(* Logix 5000 AddOnInstructionDefinition export Banner_S15C_B21_Param_v4; software revision 33.00; part 2 of 2 *)
(* tags used below, declared in another part *)
   S15C : Banner_S15C_B21_v4;
   Port_Data : Banner_IOL_Port_v4;
   Port : DINT;
   Local_Control : DINT;
   Command_Being_Processed : BOOL;
   Index_Write_Inprocess : INT;
   Index_Write_Control : INT;
   Update_Archive : BOOL;
   Inprocess_Index : DINT;
(* Banner_S15C_B21_Param_v4, continued *)

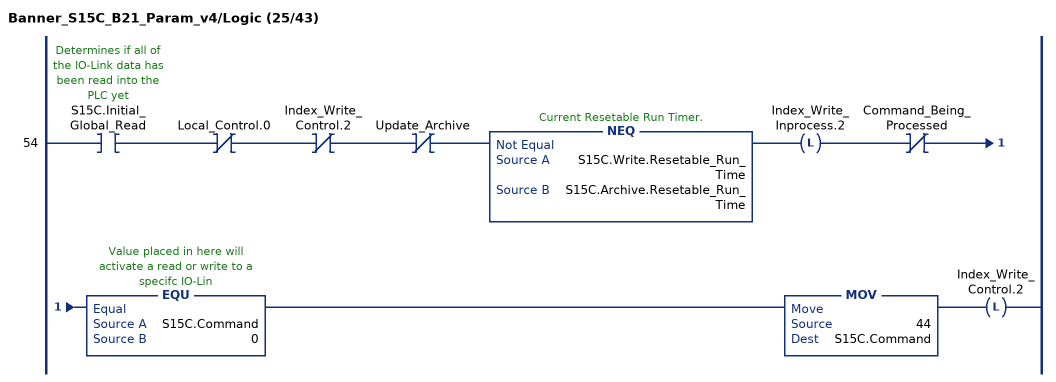
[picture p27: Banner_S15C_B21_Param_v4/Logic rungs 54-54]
   54: XIC(S15C.Initial_Global_Read)XIO(Local_Control.0)XIO(Index_Write_Control.2)XIO(Update_Archive)NEQ(S15C.Write.Resetable_Run_Time,S15C.Archive.Resetable_Run_Time)OTL(Index_Write_Inprocess.2)XIO(Command_Being_Processed)EQU(S15C.Command,0)MOV(44,S15C.Command)OTL(Index_Write_Control.2);
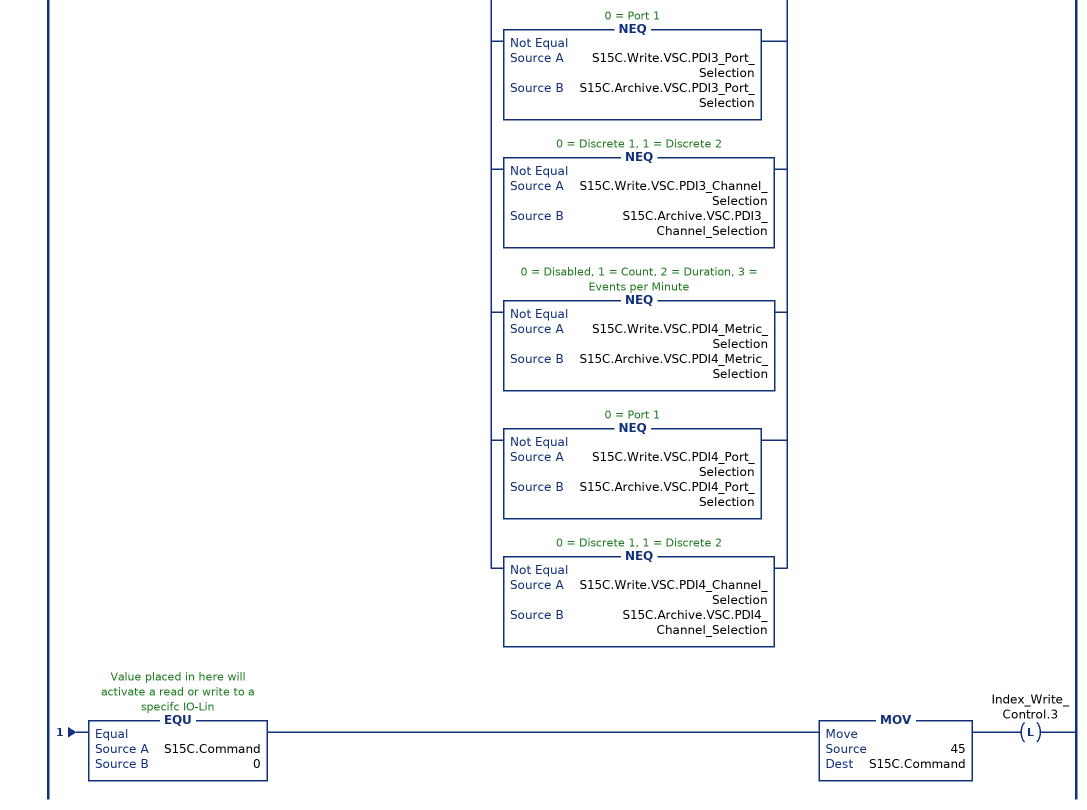
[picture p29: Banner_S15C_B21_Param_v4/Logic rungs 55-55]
   55: XIC(S15C.Initial_Global_Read)XIO(Local_Control.0)XIO(Index_Write_Control.3)XIO(Update_Archive)[NEQ(S15C.Write.VSC.PDI1_Metric_Selection,S15C.Archive.VSC.PDI1_Metric_Selection) ,NEQ(S15C.Write.VSC.PDI1_Port_Selection,S15C.Archive.VSC.PDI1_Port_Selection) ,NEQ(S15C.Write.VSC.PDI1_Channel_Selection,S15C.Archive.VSC.PDI1_Channel_Selection) ,NEQ(S15C.Write.VSC.PDI2_Metric_Selection,S15C.Archive.VSC.PDI2_Metric_Selection) ,NEQ(S15C.Write.VSC.PDI2_Port_Selection,S15C.Archive.VSC.PDI2_Port_Selection) ,NEQ(S15C.Write.VSC.PDI2_Channel_Selection,S15C.Archive.VSC.PDI2_Channel_Selection) ,NEQ(S15C.Write.VSC.PDI3_Metric_Selection,S15C.Archive.VSC.PDI3_Metric_Selection) ,NEQ(S15C.Write.VSC.PDI3_Port_Selection,S15C.Archive.VSC.PDI3_Port_Selection) ,NEQ(S15C.Write.VSC.PDI3_Channel_Selection,S15C.Archive.VSC.PDI3_Channel_Selection) ,NEQ(S15C.Write.VSC.PDI4_Metric_Selection,S15C.Archive.VSC.PDI4_Metric_Selection) ,NEQ(S15C.Write.VSC.PDI4_Port_Selection,S15C.Archive.VSC.PDI4_Port_Selection) ,NEQ(S15C.Write.VSC.PDI4_Channel_Selection,S15C.Archive.VSC.PDI4_Channel_Selection) ]OTL(Index_Write_Inprocess.3)XIO(Command_Being_Processed)EQU(S15C.Command,0)MOV(45,S15C.Command)OTL(Index_Write_Control.3);
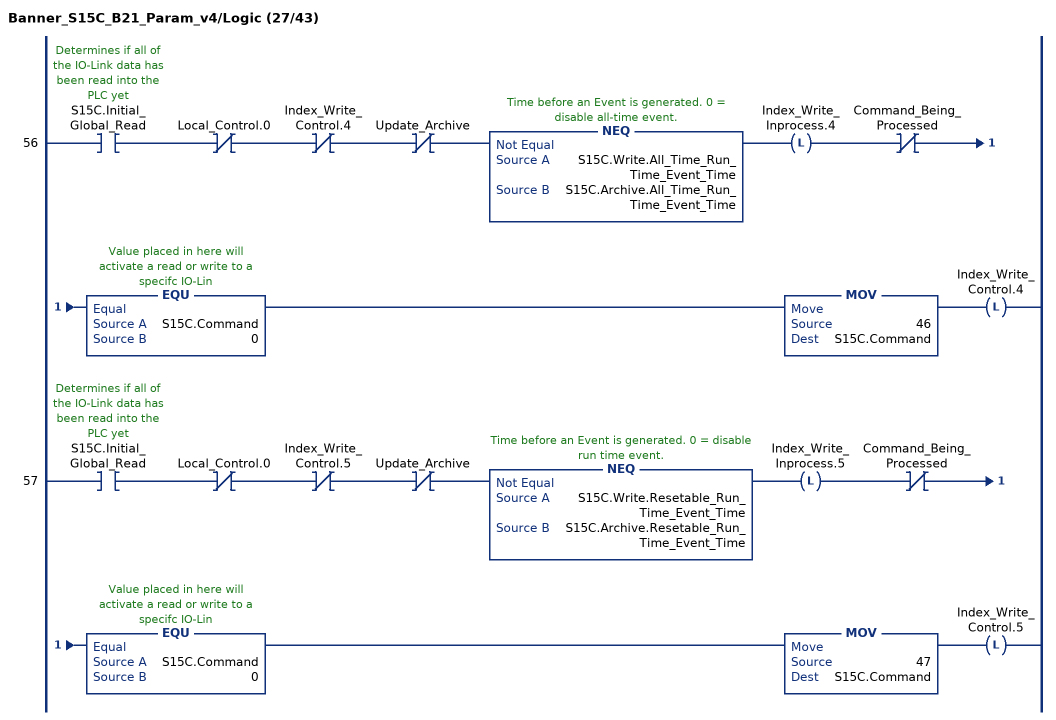
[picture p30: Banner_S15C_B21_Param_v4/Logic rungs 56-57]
   56: XIC(S15C.Initial_Global_Read)XIO(Local_Control.0)XIO(Index_Write_Control.4)XIO(Update_Archive)NEQ(S15C.Write.All_Time_Run_Time_Event_Time,S15C.Archive.All_Time_Run_Time_Event_Time)OTL(Index_Write_Inprocess.4)XIO(Command_Being_Processed)EQU(S15C.Command,0)MOV(46,S15C.Command)OTL(Index_Write_Control.4);
   57: XIC(S15C.Initial_Global_Read)XIO(Local_Control.0)XIO(Index_Write_Control.5)XIO(Update_Archive)NEQ(S15C.Write.Resetable_Run_Time_Event_Time,S15C.Archive.Resetable_Run_Time_Event_Time)OTL(Index_Write_Inprocess.5)XIO(Command_Being_Processed)EQU(S15C.Command,0)MOV(47,S15C.Command)OTL(Index_Write_Control.5);
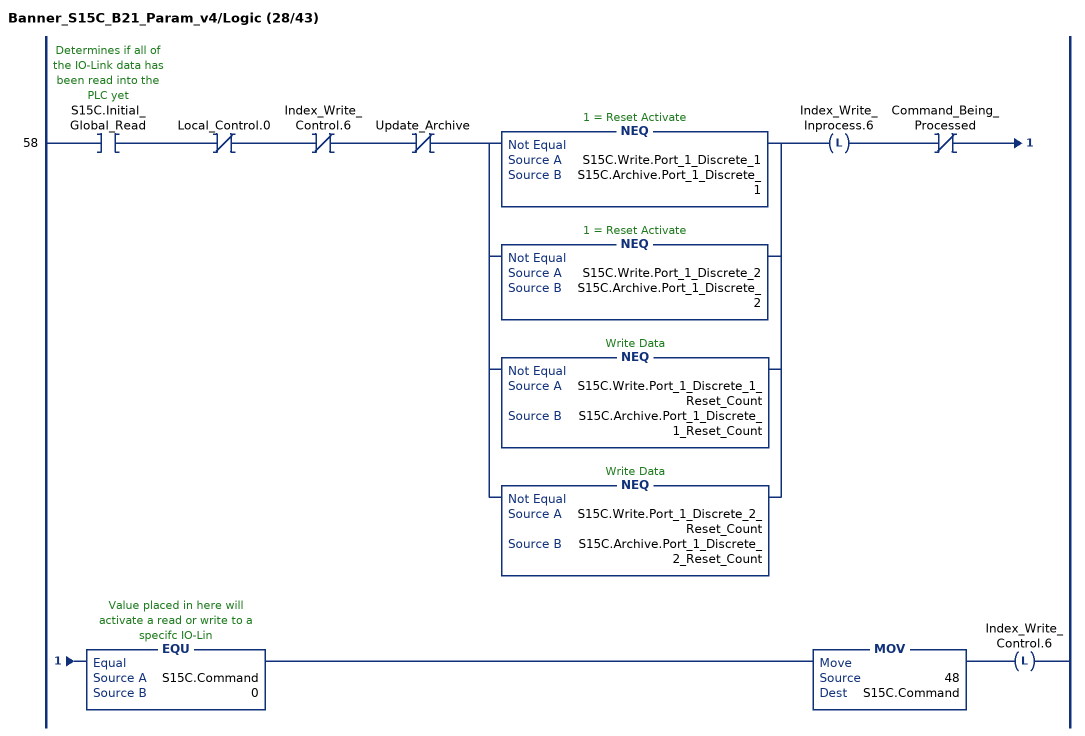
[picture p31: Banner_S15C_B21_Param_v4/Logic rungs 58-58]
   58: XIC(S15C.Initial_Global_Read)XIO(Local_Control.0)XIO(Index_Write_Control.6)XIO(Update_Archive)[NEQ(S15C.Write.Port_1_Discrete_1,S15C.Archive.Port_1_Discrete_1) ,NEQ(S15C.Write.Port_1_Discrete_2,S15C.Archive.Port_1_Discrete_2) ,NEQ(S15C.Write.Port_1_Discrete_1_Reset_Count,S15C.Archive.Port_1_Discrete_1_Reset_Count) ,NEQ(S15C.Write.Port_1_Discrete_2_Reset_Count,S15C.Archive.Port_1_Discrete_2_Reset_Count) ]OTL(Index_Write_Inprocess.6)XIO(Command_Being_Processed)EQU(S15C.Command,0)MOV(48,S15C.Command)OTL(Index_Write_Control.6);
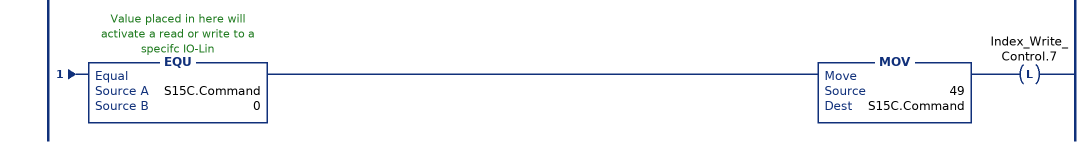
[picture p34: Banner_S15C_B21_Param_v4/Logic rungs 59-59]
   59: XIC(S15C.Initial_Global_Read)XIO(Local_Control.0)XIO(Index_Write_Control.7)XIO(Update_Archive)[NEQ(S15C.Write.Port_1_Configuration.DI1_IO_Selection,S15C.Archive.Port_1_Configuration.DI1_IO_Selection) ,NEQ(S15C.Write.Port_1_Configuration.DI1_Delay_Mode,S15C.Archive.Port_1_Configuration.DI1_Delay_Mode) ,NEQ(S15C.Write.Port_1_Configuration.DI1_Delay_Timer_1,S15C.Archive.Port_1_Configuration.DI1_Delay_Timer_1) ,NEQ(S15C.Write.Port_1_Configuration.DI1_Delay_Timer_2,S15C.Archive.Port_1_Configuration.DI1_Delay_Timer_2) ,NEQ(S15C.Write.Port_1_Configuration.DI2_IO_Selection,S15C.Archive.Port_1_Configuration.DI2_IO_Selection) ,NEQ(S15C.Write.Port_1_Configuration.DI2_Delay_Mode,S15C.Archive.Port_1_Configuration.DI2_Delay_Mode) ,NEQ(S15C.Write.Port_1_Configuration.DI2_Delay_Timer_1,S15C.Archive.Port_1_Configuration.DI2_Delay_Timer_1) ,NEQ(S15C.Write.Port_1_Configuration.DI2_Delay_Timer_2,S15C.Archive.Port_1_Configuration.DI2_Delay_Timer_2) ,NEQ(S15C.Write.Port_1_Configuration.Mirroring_Enable,S15C.Archive.Port_1_Configuration.Mirroring_Enable) ,NEQ(S15C.Write.Port_1_Configuration.Mirroring_Port_Selection,S15C.Archive.Port_1_Configuration.Mirroring_Port_Selection) ,NEQ(S15C.Write.Port_1_Configuration.Mirroring_Channel_Selection,S15C.Archive.Port_1_Configuration.Mirroring_Channel_Selection) ,NEQ(S15C.Write.Port_1_Configuration.Mirroring_Inversion,S15C.Archive.Port_1_Configuration.Mirroring_Inversion) ,NEQ(S15C.Write.Port_1_Configuration.Counts_per_Minute_Mode,S15C.Archive.Port_1_Configuration.Counts_per_Minute_Mode) ]OTL(Index_Write_Inprocess.7)XIO(Command_Being_Processed)EQU(S15C.Command,0)MOV(49,S15C.Command)OTL(Index_Write_Control.7);
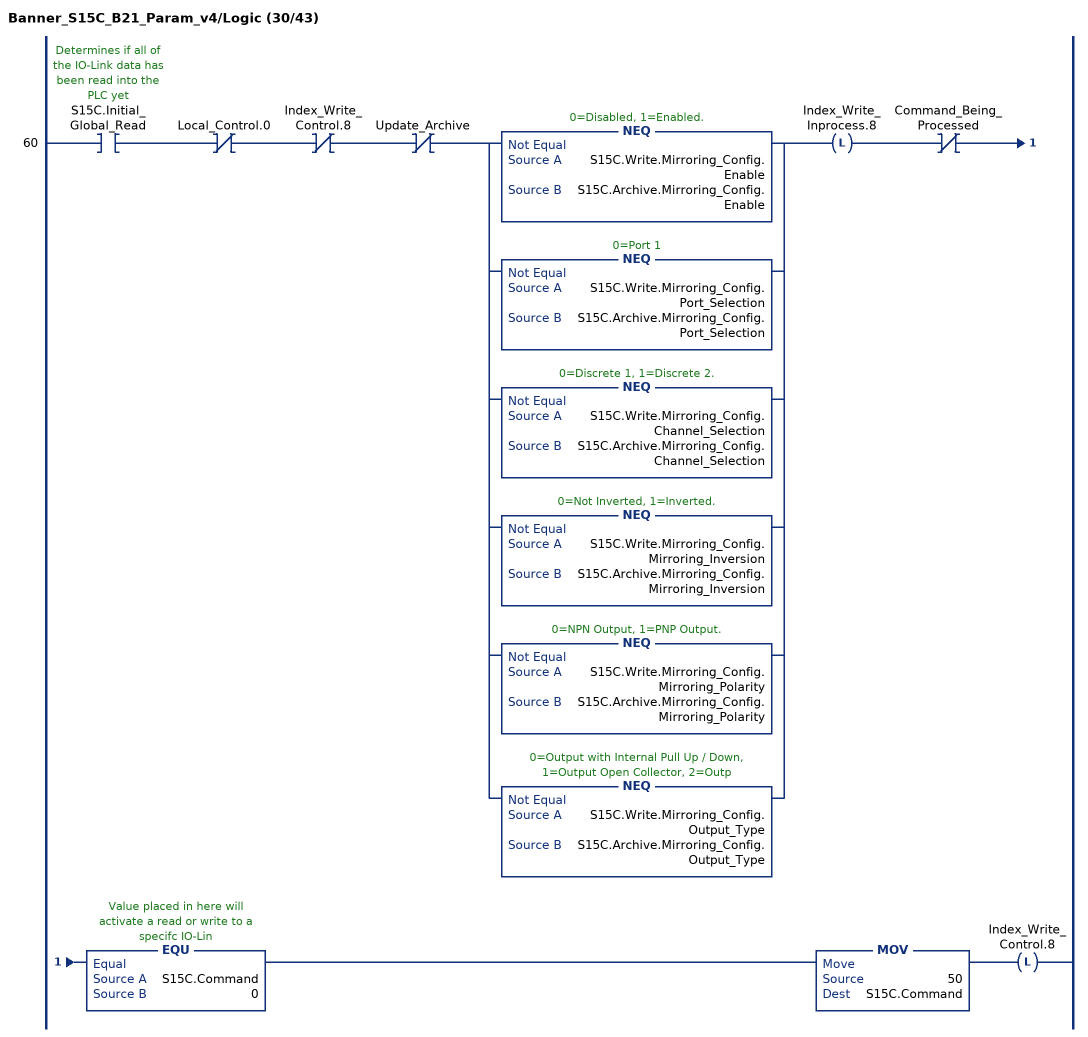
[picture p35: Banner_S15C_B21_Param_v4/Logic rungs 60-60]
   60: XIC(S15C.Initial_Global_Read)XIO(Local_Control.0)XIO(Index_Write_Control.8)XIO(Update_Archive)[NEQ(S15C.Write.Mirroring_Config.Enable,S15C.Archive.Mirroring_Config.Enable) ,NEQ(S15C.Write.Mirroring_Config.Port_Selection,S15C.Archive.Mirroring_Config.Port_Selection) ,NEQ(S15C.Write.Mirroring_Config.Channel_Selection,S15C.Archive.Mirroring_Config.Channel_Selection) ,NEQ(S15C.Write.Mirroring_Config.Mirroring_Inversion,S15C.Archive.Mirroring_Config.Mirroring_Inversion) ,NEQ(S15C.Write.Mirroring_Config.Mirroring_Polarity,S15C.Archive.Mirroring_Config.Mirroring_Polarity) ,NEQ(S15C.Write.Mirroring_Config.Output_Type,S15C.Archive.Mirroring_Config.Output_Type) ]OTL(Index_Write_Inprocess.8)XIO(Command_Being_Processed)EQU(S15C.Command,0)MOV(50,S15C.Command)OTL(Index_Write_Control.8);
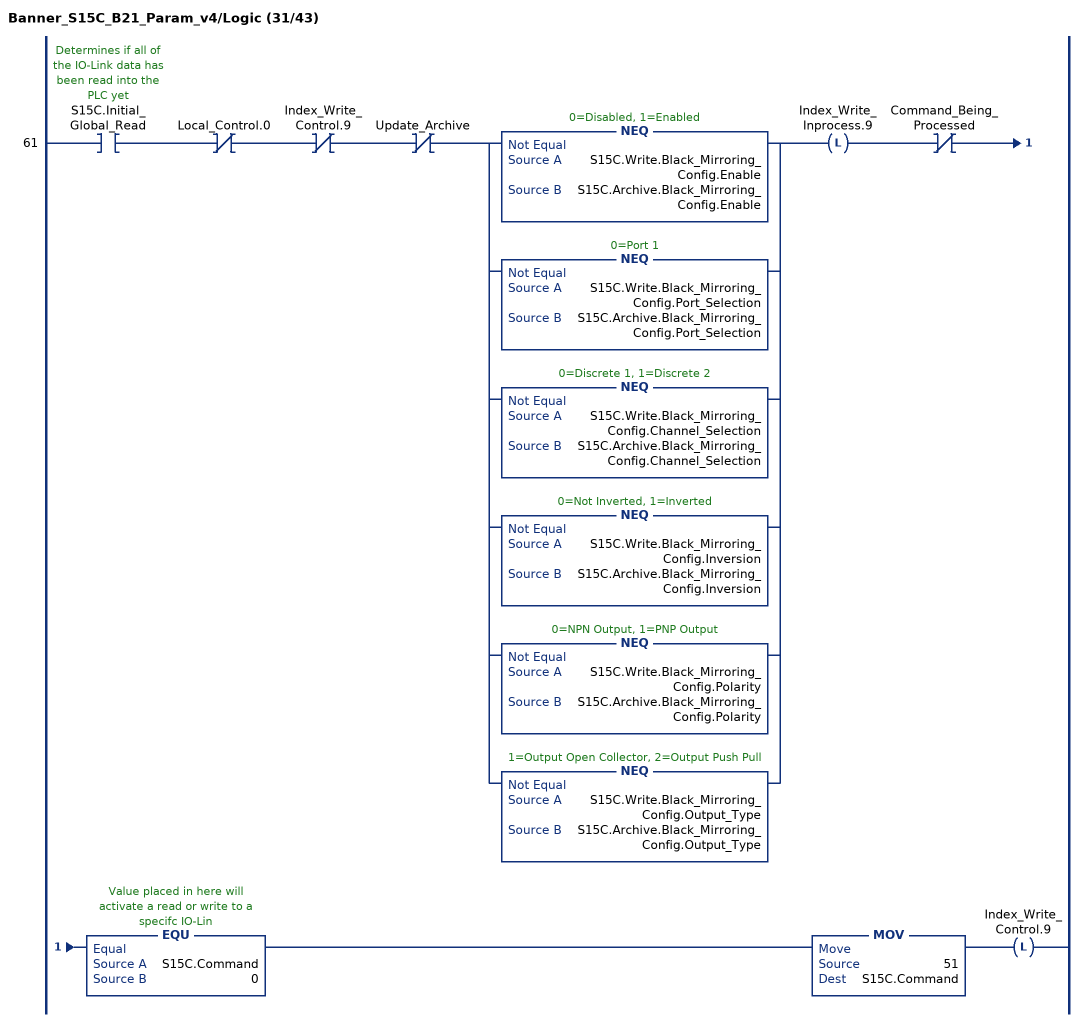
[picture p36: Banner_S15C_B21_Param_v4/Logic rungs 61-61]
   61: XIC(S15C.Initial_Global_Read)XIO(Local_Control.0)XIO(Index_Write_Control.9)XIO(Update_Archive)[NEQ(S15C.Write.Black_Mirroring_Config.Enable,S15C.Archive.Black_Mirroring_Config.Enable) ,NEQ(S15C.Write.Black_Mirroring_Config.Port_Selection,S15C.Archive.Black_Mirroring_Config.Port_Selection) ,NEQ(S15C.Write.Black_Mirroring_Config.Channel_Selection,S15C.Archive.Black_Mirroring_Config.Channel_Selection) ,NEQ(S15C.Write.Black_Mirroring_Config.Inversion,S15C.Archive.Black_Mirroring_Config.Inversion) ,NEQ(S15C.Write.Black_Mirroring_Config.Polarity,S15C.Archive.Black_Mirroring_Config.Polarity) ,NEQ(S15C.Write.Black_Mirroring_Config.Output_Type,S15C.Archive.Black_Mirroring_Config.Output_Type) ]OTL(Index_Write_Inprocess.9)XIO(Command_Being_Processed)EQU(S15C.Command,0)MOV(51,S15C.Command)OTL(Index_Write_Control.9);
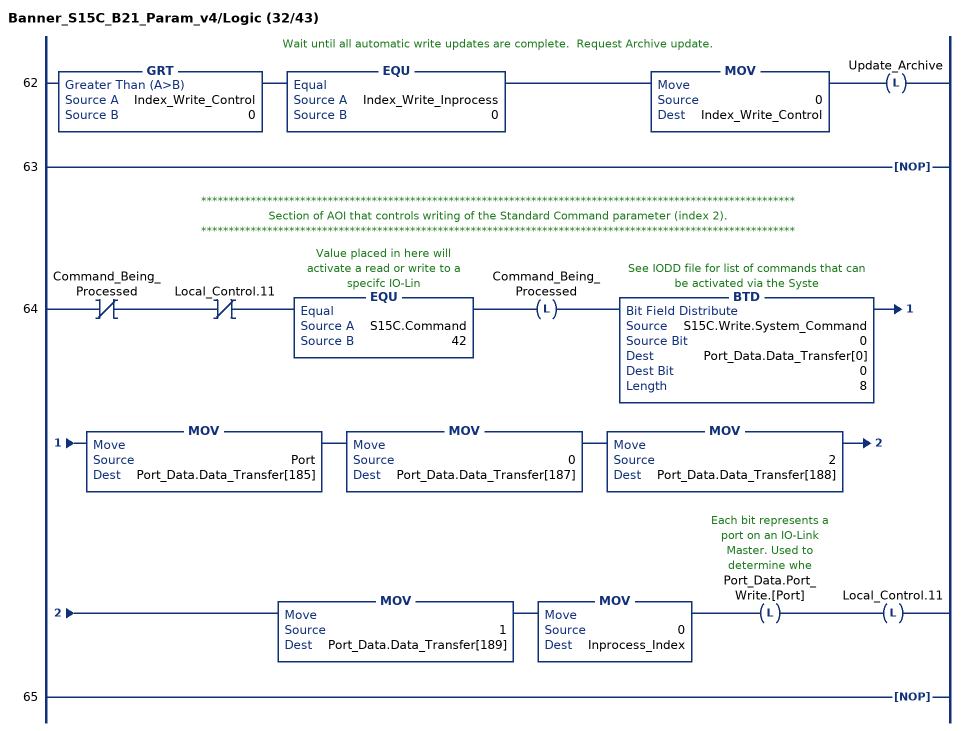
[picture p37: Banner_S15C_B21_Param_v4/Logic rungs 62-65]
   // Wait until all automatic write updates are complete.  Request Archive update.
   62: GRT(Index_Write_Control,0)EQU(Index_Write_Inprocess,0)MOV(0,Index_Write_Control)OTL(Update_Archive);
   63: NOP();
   // ************************************************************************************************************
   // Section of AOI that controls writing of the Standard Command parameter (index 2).
   // ************************************************************************************************************
   64: XIO(Command_Being_Processed)XIO(Local_Control.11)EQU(S15C.Command,42)OTL(Command_Being_Processed)BTD(S15C.Write.System_Command,0,Port_Data.Data_Transfer[0],0,8)MOV(Port,Port_Data.Data_Transfer[185])MOV(0,Port_Data.Data_Transfer[187])MOV(2,Port_Data.Data_Transfer[188])MOV(1,Port_Data.Data_Transfer[189])MOV(0,Inprocess_Index)OTL(Port_Data.Port_Write.[Port])OTL(Local_Control.11);
   65: NOP();
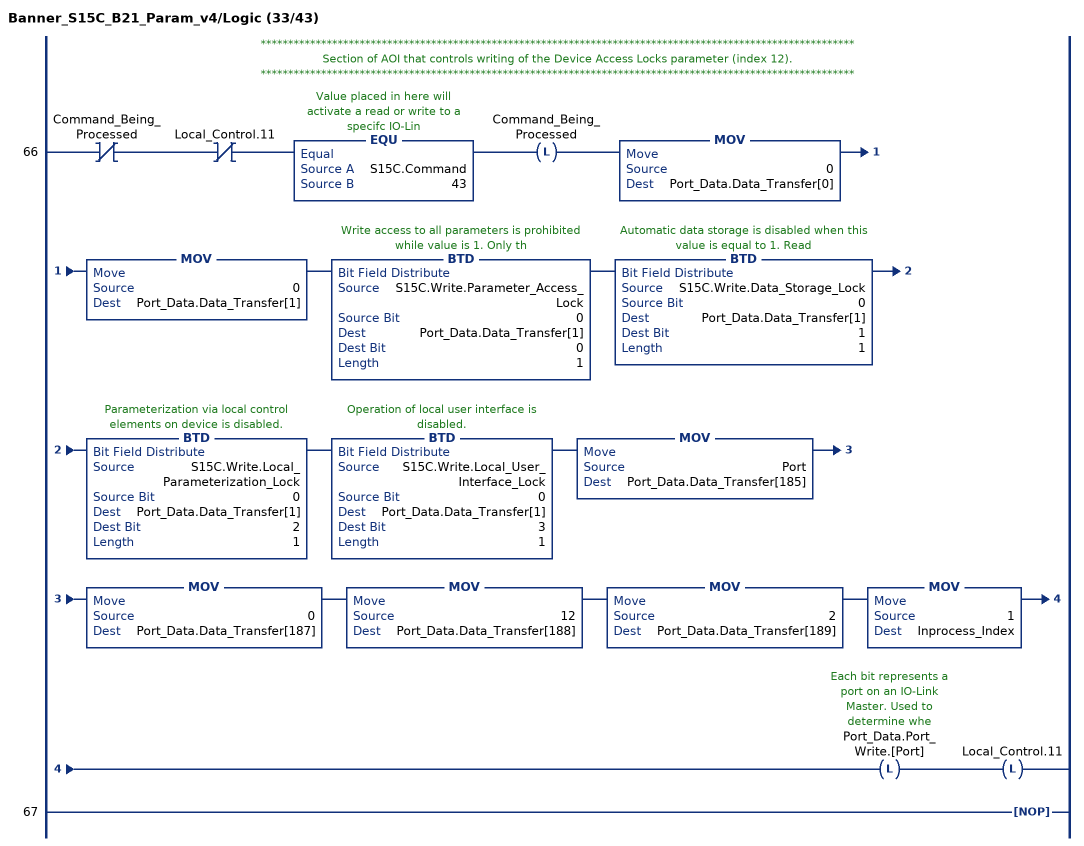
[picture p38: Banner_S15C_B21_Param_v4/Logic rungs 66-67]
   // ************************************************************************************************************
   // Section of AOI that controls writing of the Device Access Locks parameter (index 12).
   // ************************************************************************************************************
   66: XIO(Command_Being_Processed)XIO(Local_Control.11)EQU(S15C.Command,43)OTL(Command_Being_Processed)MOV(0,Port_Data.Data_Transfer[0])MOV(0,Port_Data.Data_Transfer[1])BTD(S15C.Write.Parameter_Access_Lock,0,Port_Data.Data_Transfer[1],0,1)BTD(S15C.Write.Data_Storage_Lock,0,Port_Data.Data_Transfer[1],1,1)BTD(S15C.Write.Local_Parameterization_Lock,0,Port_Data.Data_Transfer[1],2,1)BTD(S15C.Write.Local_User_Interface_Lock,0,Port_Data.Data_Transfer[1],3,1)MOV(Port,Port_Data.Data_Transfer[185])MOV(0,Port_Data.Data_Transfer[187])MOV(12,Port_Data.Data_Transfer[188])MOV(2,Port_Data.Data_Transfer[189])MOV(1,Inprocess_Index)OTL(Port_Data.Port_Write.[Port])OTL(Local_Control.11);
   67: NOP();
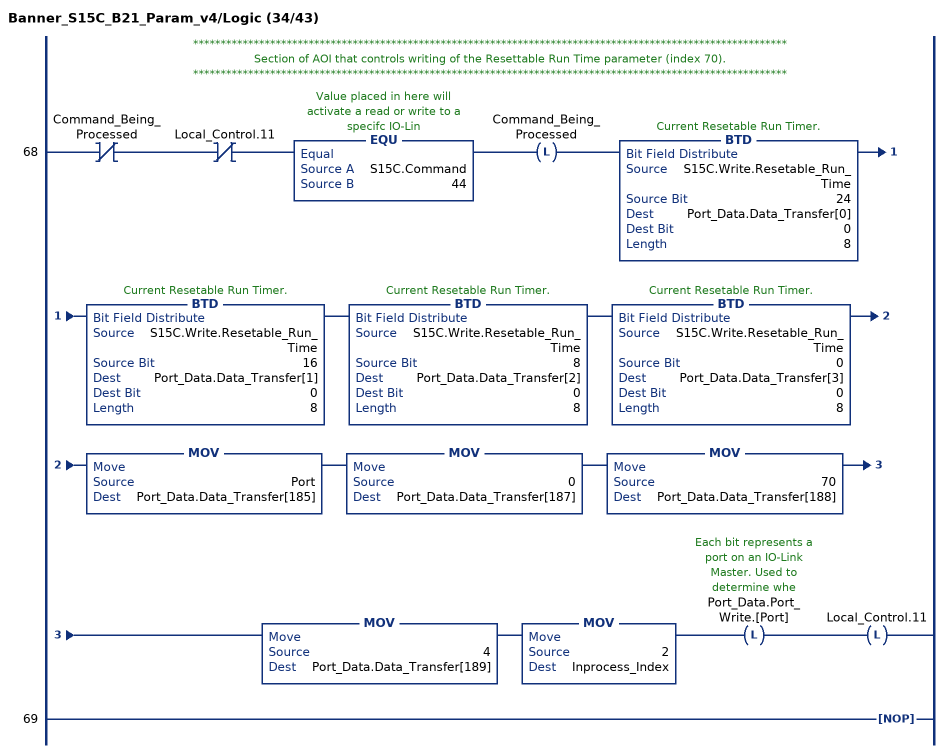
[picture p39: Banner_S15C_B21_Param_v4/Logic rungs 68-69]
   // ************************************************************************************************************
   // Section of AOI that controls writing of the Resettable Run Time parameter (index 70).
   // ************************************************************************************************************
   68: XIO(Command_Being_Processed)XIO(Local_Control.11)EQU(S15C.Command,44)OTL(Command_Being_Processed)BTD(S15C.Write.Resetable_Run_Time,24,Port_Data.Data_Transfer[0],0,8)BTD(S15C.Write.Resetable_Run_Time,16,Port_Data.Data_Transfer[1],0,8)BTD(S15C.Write.Resetable_Run_Time,8,Port_Data.Data_Transfer[2],0,8)BTD(S15C.Write.Resetable_Run_Time,0,Port_Data.Data_Transfer[3],0,8)MOV(Port,Port_Data.Data_Transfer[185])MOV(0,Port_Data.Data_Transfer[187])MOV(70,Port_Data.Data_Transfer[188])MOV(4,Port_Data.Data_Transfer[189])MOV(2,Inprocess_Index)OTL(Port_Data.Port_Write.[Port])OTL(Local_Control.11);
   69: NOP();
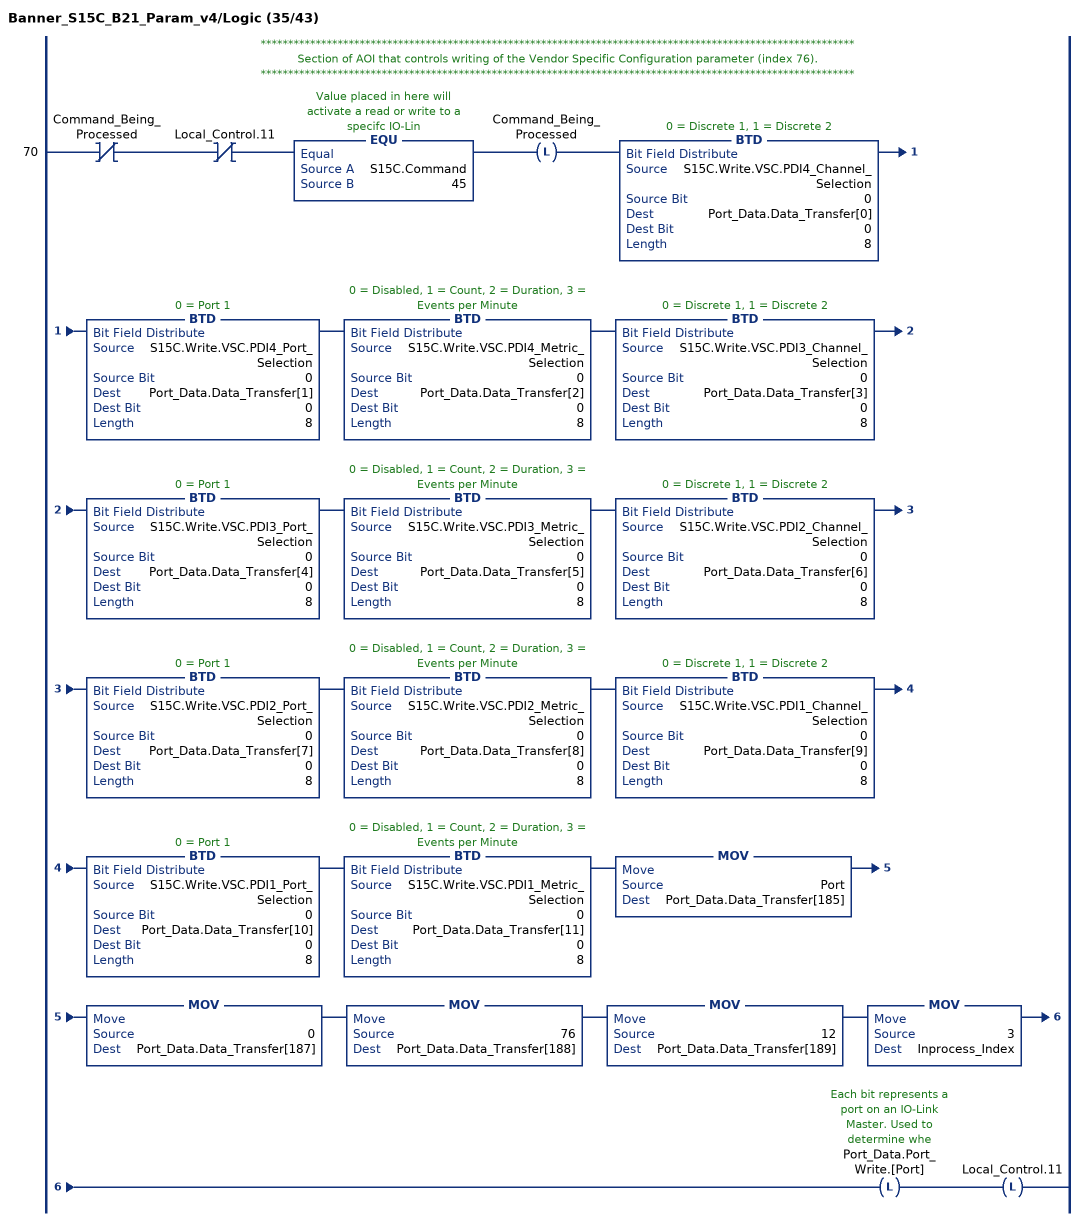
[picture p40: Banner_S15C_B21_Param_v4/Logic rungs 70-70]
   // ************************************************************************************************************
   // Section of AOI that controls writing of the Vendor Specific Configuration parameter (index 76).
   // ************************************************************************************************************
   70: XIO(Command_Being_Processed)XIO(Local_Control.11)EQU(S15C.Command,45)OTL(Command_Being_Processed)BTD(S15C.Write.VSC.PDI4_Channel_Selection,0,Port_Data.Data_Transfer[0],0,8)BTD(S15C.Write.VSC.PDI4_Port_Selection,0,Port_Data.Data_Transfer[1],0,8)BTD(S15C.Write.VSC.PDI4_Metric_Selection,0,Port_Data.Data_Transfer[2],0,8)BTD(S15C.Write.VSC.PDI3_Channel_Selection,0,Port_Data.Data_Transfer[3],0,8)BTD(S15C.Write.VSC.PDI3_Port_Selection,0,Port_Data.Data_Transfer[4],0,8)BTD(S15C.Write.VSC.PDI3_Metric_Selection,0,Port_Data.Data_Transfer[5],0,8)BTD(S15C.Write.VSC.PDI2_Channel_Selection,0,Port_Data.Data_Transfer[6],0,8)BTD(S15C.Write.VSC.PDI2_Port_Selection,0,Port_Data.Data_Transfer[7],0,8)BTD(S15C.Write.VSC.PDI2_Metric_Selection,0,Port_Data.Data_Transfer[8],0,8)BTD(S15C.Write.VSC.PDI1_Channel_Selection,0,Port_Data.Data_Transfer[9],0,8)BTD(S15C.Write.VSC.PDI1_Port_Selection,0,Port_Data.Data_Transfer[10],0,8)BTD(S15C.Write.VSC.PDI1_Metric_Selection,0,Port_Data.Data_Transfer[11],0,8)MOV(Port,Port_Data.Data_Transfer[185])MOV(0,Port_Data.Data_Transfer[187])MOV(76,Port_Data.Data_Transfer[188])MOV(12,Port_Data.Data_Transfer[189])MOV(3,Inprocess_Index)OTL(Port_Data.Port_Write.[Port])OTL(Local_Control.11);
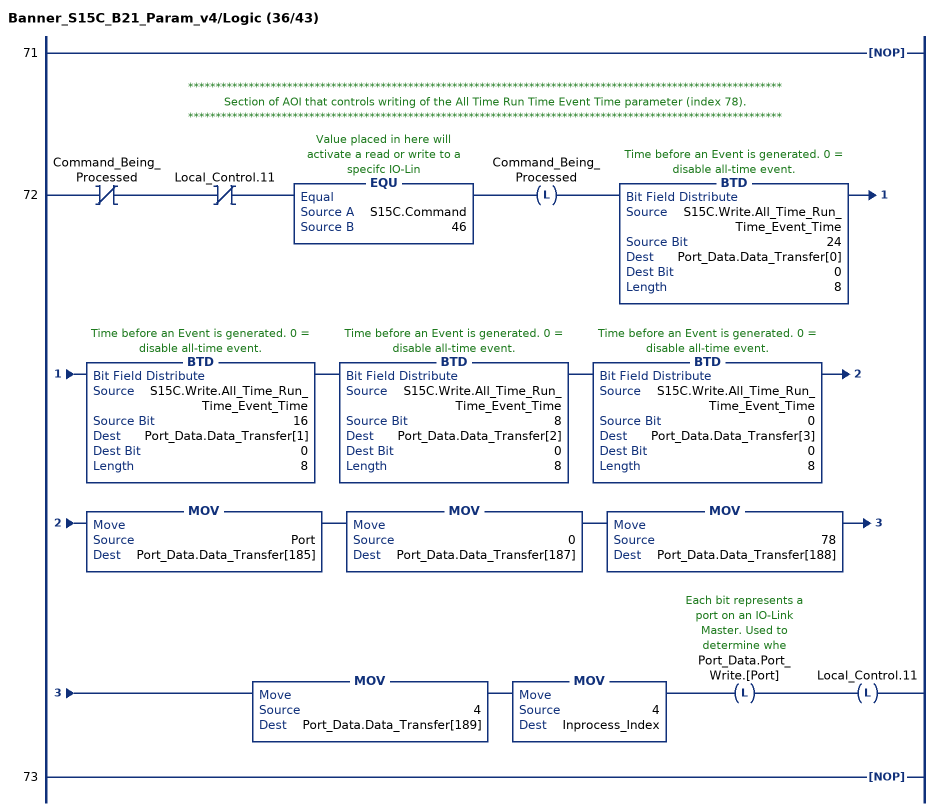
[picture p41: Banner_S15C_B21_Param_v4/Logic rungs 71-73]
   71: NOP();
   // ************************************************************************************************************
   // Section of AOI that controls writing of the All Time Run Time Event Time parameter (index 78).
   // ************************************************************************************************************
   72: XIO(Command_Being_Processed)XIO(Local_Control.11)EQU(S15C.Command,46)OTL(Command_Being_Processed)BTD(S15C.Write.All_Time_Run_Time_Event_Time,24,Port_Data.Data_Transfer[0],0,8)BTD(S15C.Write.All_Time_Run_Time_Event_Time,16,Port_Data.Data_Transfer[1],0,8)BTD(S15C.Write.All_Time_Run_Time_Event_Time,8,Port_Data.Data_Transfer[2],0,8)BTD(S15C.Write.All_Time_Run_Time_Event_Time,0,Port_Data.Data_Transfer[3],0,8)MOV(Port,Port_Data.Data_Transfer[185])MOV(0,Port_Data.Data_Transfer[187])MOV(78,Port_Data.Data_Transfer[188])MOV(4,Port_Data.Data_Transfer[189])MOV(4,Inprocess_Index)OTL(Port_Data.Port_Write.[Port])OTL(Local_Control.11);
   73: NOP();
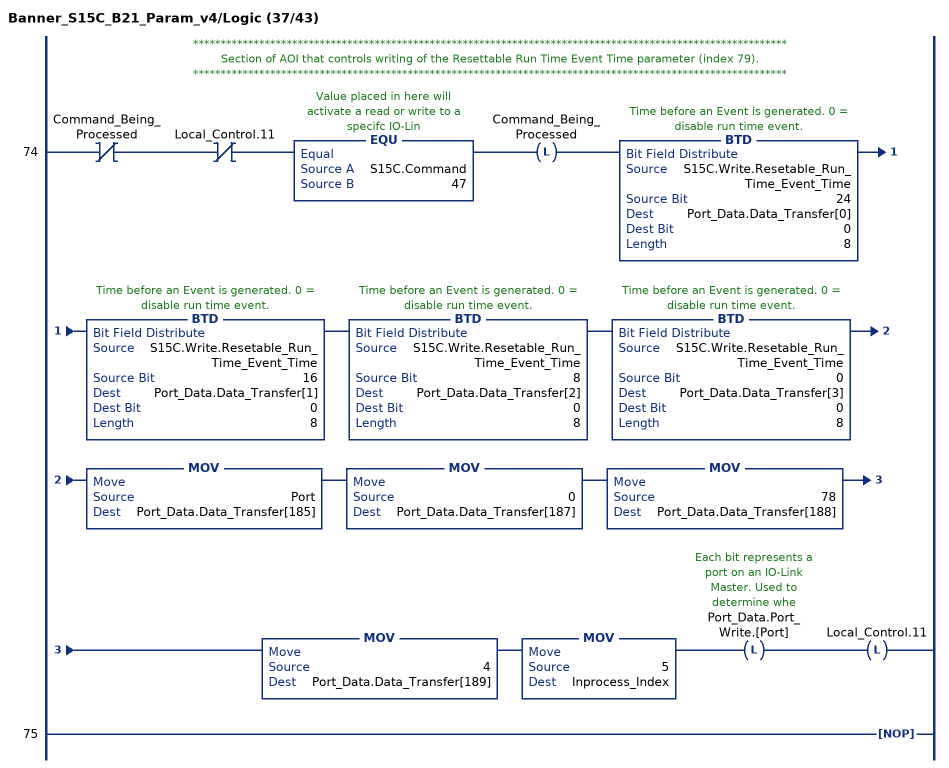
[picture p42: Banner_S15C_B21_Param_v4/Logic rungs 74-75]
   // ************************************************************************************************************
   // Section of AOI that controls writing of the Resettable Run Time Event Time parameter (index 79).
   // ************************************************************************************************************
   74: XIO(Command_Being_Processed)XIO(Local_Control.11)EQU(S15C.Command,47)OTL(Command_Being_Processed)BTD(S15C.Write.Resetable_Run_Time_Event_Time,24,Port_Data.Data_Transfer[0],0,8)BTD(S15C.Write.Resetable_Run_Time_Event_Time,16,Port_Data.Data_Transfer[1],0,8)BTD(S15C.Write.Resetable_Run_Time_Event_Time,8,Port_Data.Data_Transfer[2],0,8)BTD(S15C.Write.Resetable_Run_Time_Event_Time,0,Port_Data.Data_Transfer[3],0,8)MOV(Port,Port_Data.Data_Transfer[185])MOV(0,Port_Data.Data_Transfer[187])MOV(78,Port_Data.Data_Transfer[188])MOV(4,Port_Data.Data_Transfer[189])MOV(5,Inprocess_Index)OTL(Port_Data.Port_Write.[Port])OTL(Local_Control.11);
   75: NOP();
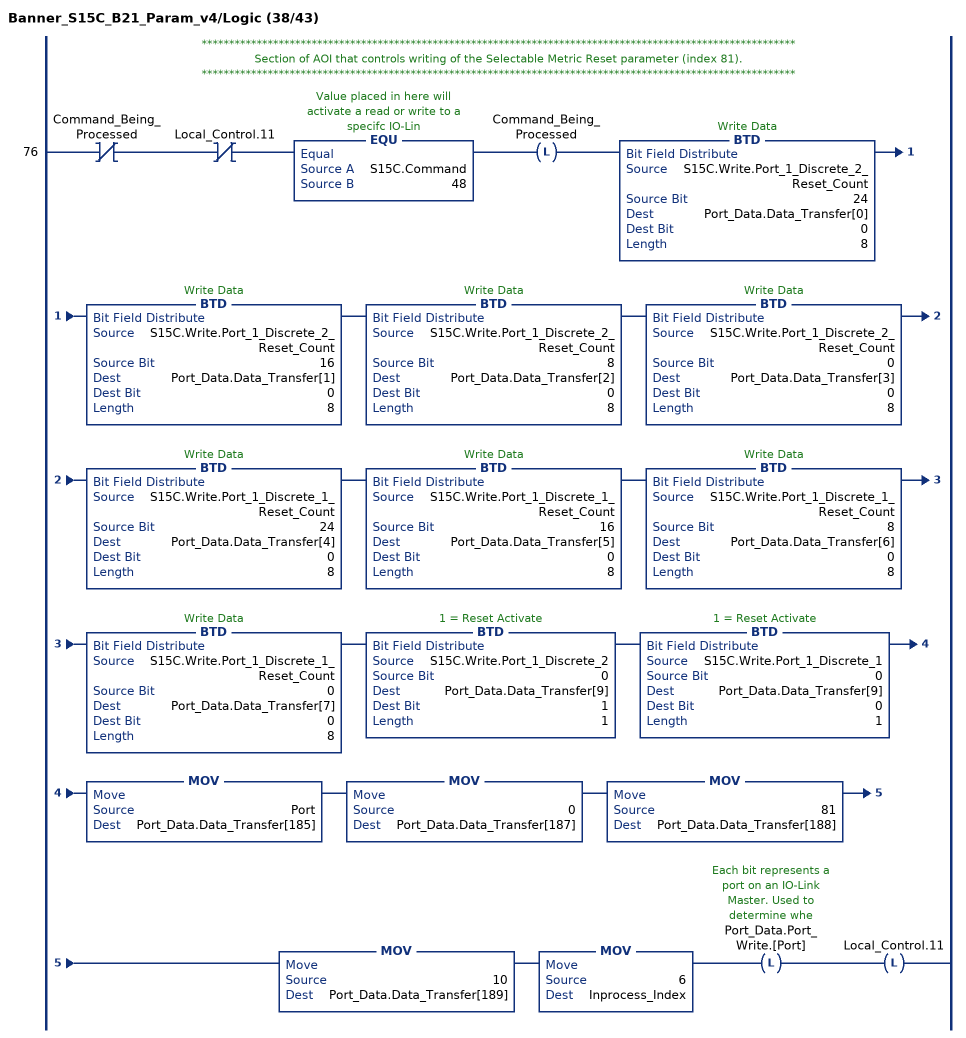
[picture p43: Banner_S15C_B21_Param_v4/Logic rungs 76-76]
   // ************************************************************************************************************
   // Section of AOI that controls writing of the Selectable Metric Reset parameter (index 81).
   // ************************************************************************************************************
   76: XIO(Command_Being_Processed)XIO(Local_Control.11)EQU(S15C.Command,48)OTL(Command_Being_Processed)BTD(S15C.Write.Port_1_Discrete_2_Reset_Count,24,Port_Data.Data_Transfer[0],0,8)BTD(S15C.Write.Port_1_Discrete_2_Reset_Count,16,Port_Data.Data_Transfer[1],0,8)BTD(S15C.Write.Port_1_Discrete_2_Reset_Count,8,Port_Data.Data_Transfer[2],0,8)BTD(S15C.Write.Port_1_Discrete_2_Reset_Count,0,Port_Data.Data_Transfer[3],0,8)BTD(S15C.Write.Port_1_Discrete_1_Reset_Count,24,Port_Data.Data_Transfer[4],0,8)BTD(S15C.Write.Port_1_Discrete_1_Reset_Count,16,Port_Data.Data_Transfer[5],0,8)BTD(S15C.Write.Port_1_Discrete_1_Reset_Count,8,Port_Data.Data_Transfer[6],0,8)BTD(S15C.Write.Port_1_Discrete_1_Reset_Count,0,Port_Data.Data_Transfer[7],0,8)BTD(S15C.Write.Port_1_Discrete_2,0,Port_Data.Data_Transfer[9],1,1)BTD(S15C.Write.Port_1_Discrete_1,0,Port_Data.Data_Transfer[9],0,1)MOV(Port,Port_Data.Data_Transfer[185])MOV(0,Port_Data.Data_Transfer[187])MOV(81,Port_Data.Data_Transfer[188])MOV(10,Port_Data.Data_Transfer[189])MOV(6,Inprocess_Index)OTL(Port_Data.Port_Write.[Port])OTL(Local_Control.11);
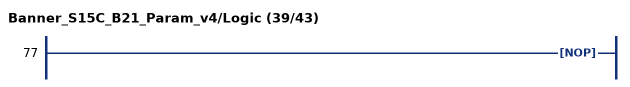
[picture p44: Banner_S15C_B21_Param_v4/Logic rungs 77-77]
   77: NOP();
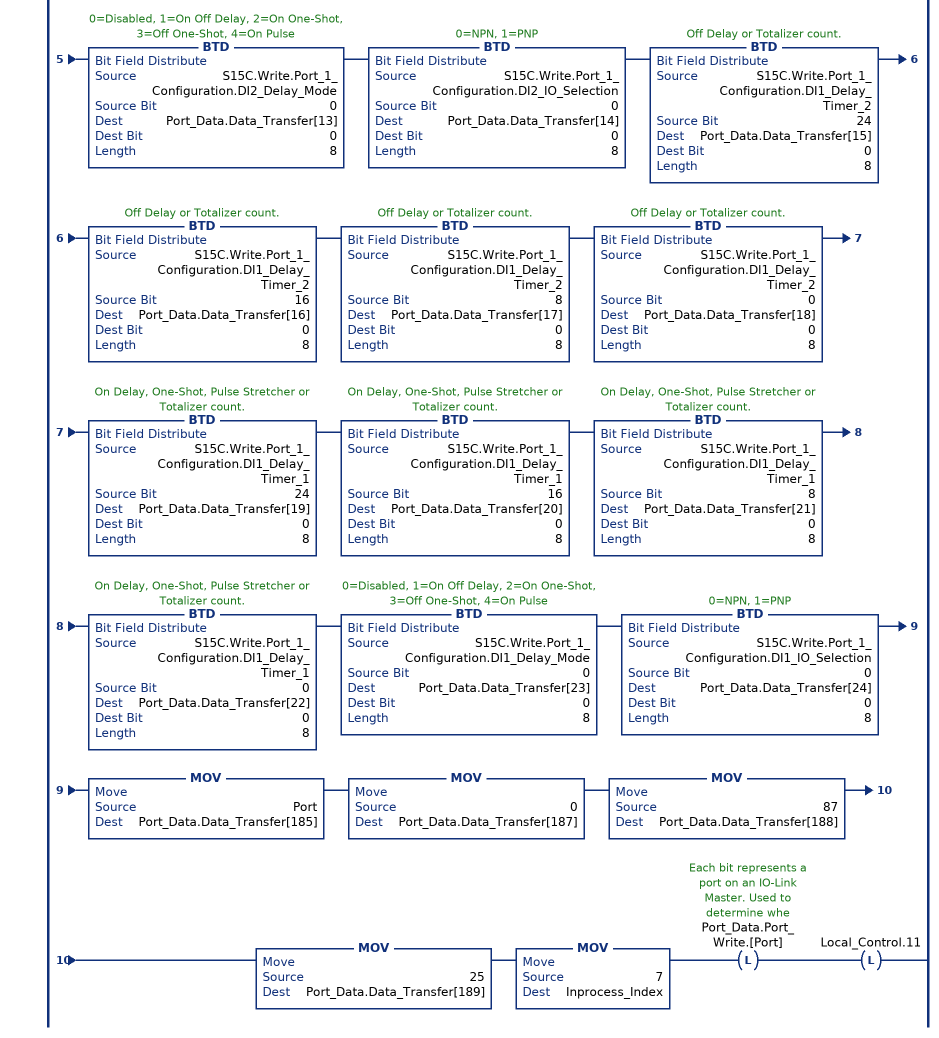
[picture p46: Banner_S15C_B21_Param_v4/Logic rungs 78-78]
   // ************************************************************************************************************
   // Section of AOI that controls writing of the Port Configuration parameter (index 87).
   // ************************************************************************************************************
   78: XIO(Command_Being_Processed)XIO(Local_Control.11)EQU(S15C.Command,49)OTL(Command_Being_Processed)BTD(S15C.Write.Port_1_Configuration.Counts_per_Minute_Mode,0,Port_Data.Data_Transfer[0],0,8)BTD(S15C.Write.Port_1_Configuration.Mirroring_Inversion,0,Port_Data.Data_Transfer[1],0,8)BTD(S15C.Write.Port_1_Configuration.Mirroring_Channel_Selection,0,Port_Data.Data_Transfer[2],0,8)BTD(S15C.Write.Port_1_Configuration.Mirroring_Port_Selection,0,Port_Data.Data_Transfer[3],0,8)BTD(S15C.Write.Port_1_Configuration.Mirroring_Enable,0,Port_Data.Data_Transfer[4],0,8)BTD(S15C.Write.Port_1_Configuration.DI2_Delay_Timer_2,24,Port_Data.Data_Transfer[5],0,8)BTD(S15C.Write.Port_1_Configuration.DI2_Delay_Timer_2,16,Port_Data.Data_Transfer[6],0,8)BTD(S15C.Write.Port_1_Configuration.DI2_Delay_Timer_2,8,Port_Data.Data_Transfer[7],0,8)BTD(S15C.Write.Port_1_Configuration.DI2_Delay_Timer_2,0,Port_Data.Data_Transfer[8],0,8)BTD(S15C.Write.Port_1_Configuration.DI2_Delay_Timer_1,24,Port_Data.Data_Transfer[9],0,8)BTD(S15C.Write.Port_1_Configuration.DI2_Delay_Timer_1,16,Port_Data.Data_Transfer[10],0,8)BTD(S15C.Write.Port_1_Configuration.DI2_Delay_Timer_1,8,Port_Data.Data_Transfer[11],0,8)BTD(S15C.Write.Port_1_Configuration.DI2_Delay_Timer_1,0,Port_Data.Data_Transfer[12],0,8)BTD(S15C.Write.Port_1_Configuration.DI2_Delay_Mode,0,Port_Data.Data_Transfer[13],0,8)BTD(S15C.Write.Port_1_Configuration.DI2_IO_Selection,0,Port_Data.Data_Transfer[14],0,8)BTD(S15C.Write.Port_1_Configuration.DI1_Delay_Timer_2,24,Port_Data.Data_Transfer[15],0,8)BTD(S15C.Write.Port_1_Configuration.DI1_Delay_Timer_2,16,Port_Data.Data_Transfer[16],0,8)BTD(S15C.Write.Port_1_Configuration.DI1_Delay_Timer_2,8,Port_Data.Data_Transfer[17],0,8)BTD(S15C.Write.Port_1_Configuration.DI1_Delay_Timer_2,0,Port_Data.Data_Transfer[18],0,8)BTD(S15C.Write.Port_1_Configuration.DI1_Delay_Timer_1,24,Port_Data.Data_Transfer[19],0,8)BTD(S15C.Write.Port_1_Configuration.DI1_Delay_Timer_1,16,Port_Data.Data_Transfer[20],0,8)BTD(S15C.Write.Port_1_Configuration.DI1_Delay_Timer_1,8,Port_Data.Data_Transfer[21],0,8)BTD(S15C.Write.Port_1_Configuration.DI1_Delay_Timer_1,0,Port_Data.Data_Transfer[22],0,8)BTD(S15C.Write.Port_1_Configuration.DI1_Delay_Mode,0,Port_Data.Data_Transfer[23],0,8)BTD(S15C.Write.Port_1_Configuration.DI1_IO_Selection,0,Port_Data.Data_Transfer[24],0,8)MOV(Port,Port_Data.Data_Transfer[185])MOV(0,Port_Data.Data_Transfer[187])MOV(87,Port_Data.Data_Transfer[188])MOV(25,Port_Data.Data_Transfer[189])MOV(7,Inprocess_Index)OTL(Port_Data.Port_Write.[Port])OTL(Local_Control.11);
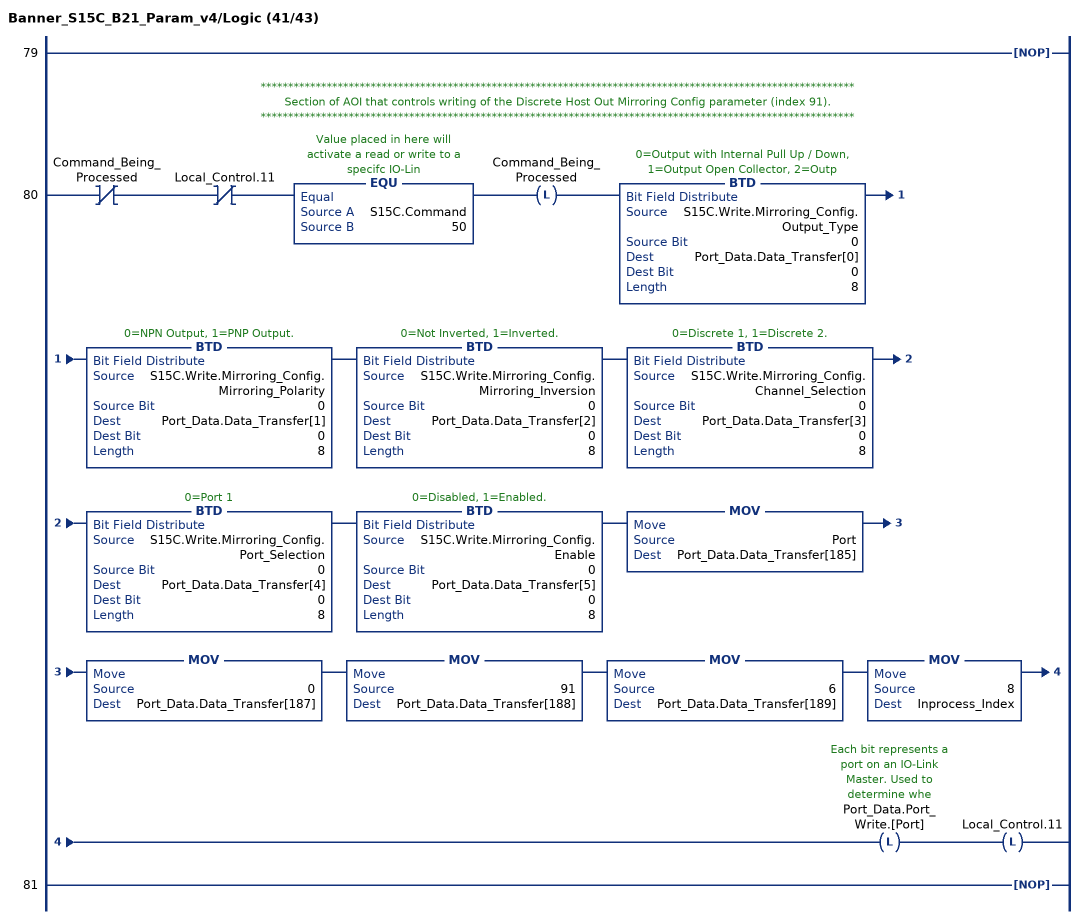
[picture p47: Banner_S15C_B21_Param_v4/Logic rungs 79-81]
   79: NOP();
   // ************************************************************************************************************
   // Section of AOI that controls writing of the Discrete Host Out Mirroring Config parameter (index 91).
   // ************************************************************************************************************
   80: XIO(Command_Being_Processed)XIO(Local_Control.11)EQU(S15C.Command,50)OTL(Command_Being_Processed)BTD(S15C.Write.Mirroring_Config.Output_Type,0,Port_Data.Data_Transfer[0],0,8)BTD(S15C.Write.Mirroring_Config.Mirroring_Polarity,0,Port_Data.Data_Transfer[1],0,8)BTD(S15C.Write.Mirroring_Config.Mirroring_Inversion,0,Port_Data.Data_Transfer[2],0,8)BTD(S15C.Write.Mirroring_Config.Channel_Selection,0,Port_Data.Data_Transfer[3],0,8)BTD(S15C.Write.Mirroring_Config.Port_Selection,0,Port_Data.Data_Transfer[4],0,8)BTD(S15C.Write.Mirroring_Config.Enable,0,Port_Data.Data_Transfer[5],0,8)MOV(Port,Port_Data.Data_Transfer[185])MOV(0,Port_Data.Data_Transfer[187])MOV(91,Port_Data.Data_Transfer[188])MOV(6,Port_Data.Data_Transfer[189])MOV(8,Inprocess_Index)OTL(Port_Data.Port_Write.[Port])OTL(Local_Control.11);
   81: NOP();
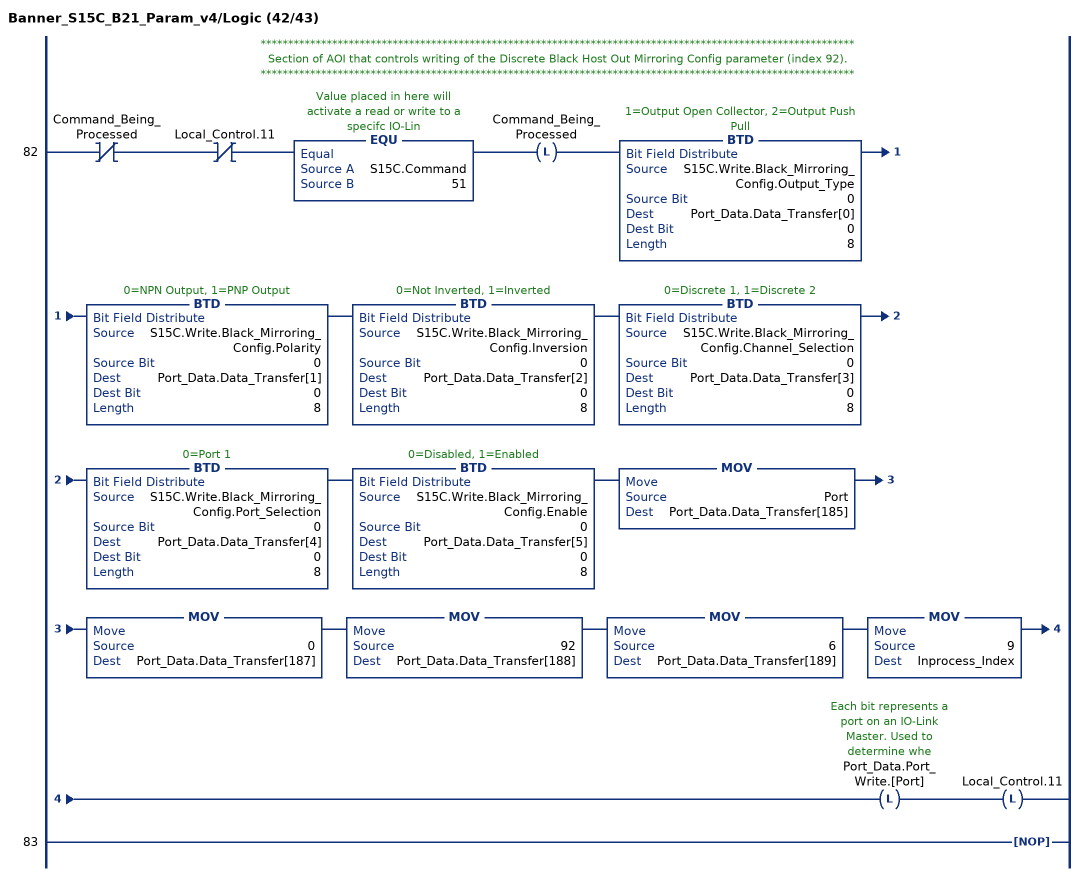
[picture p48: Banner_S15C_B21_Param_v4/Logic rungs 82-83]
   // ************************************************************************************************************
   // Section of AOI that controls writing of the Discrete Black Host Out Mirroring Config parameter (index 92).
   // ************************************************************************************************************
   82: XIO(Command_Being_Processed)XIO(Local_Control.11)EQU(S15C.Command,51)OTL(Command_Being_Processed)BTD(S15C.Write.Black_Mirroring_Config.Output_Type,0,Port_Data.Data_Transfer[0],0,8)BTD(S15C.Write.Black_Mirroring_Config.Polarity,0,Port_Data.Data_Transfer[1],0,8)BTD(S15C.Write.Black_Mirroring_Config.Inversion,0,Port_Data.Data_Transfer[2],0,8)BTD(S15C.Write.Black_Mirroring_Config.Channel_Selection,0,Port_Data.Data_Transfer[3],0,8)BTD(S15C.Write.Black_Mirroring_Config.Port_Selection,0,Port_Data.Data_Transfer[4],0,8)BTD(S15C.Write.Black_Mirroring_Config.Enable,0,Port_Data.Data_Transfer[5],0,8)MOV(Port,Port_Data.Data_Transfer[185])MOV(0,Port_Data.Data_Transfer[187])MOV(92,Port_Data.Data_Transfer[188])MOV(6,Port_Data.Data_Transfer[189])MOV(9,Inprocess_Index)OTL(Port_Data.Port_Write.[Port])OTL(Local_Control.11);
   83: NOP();
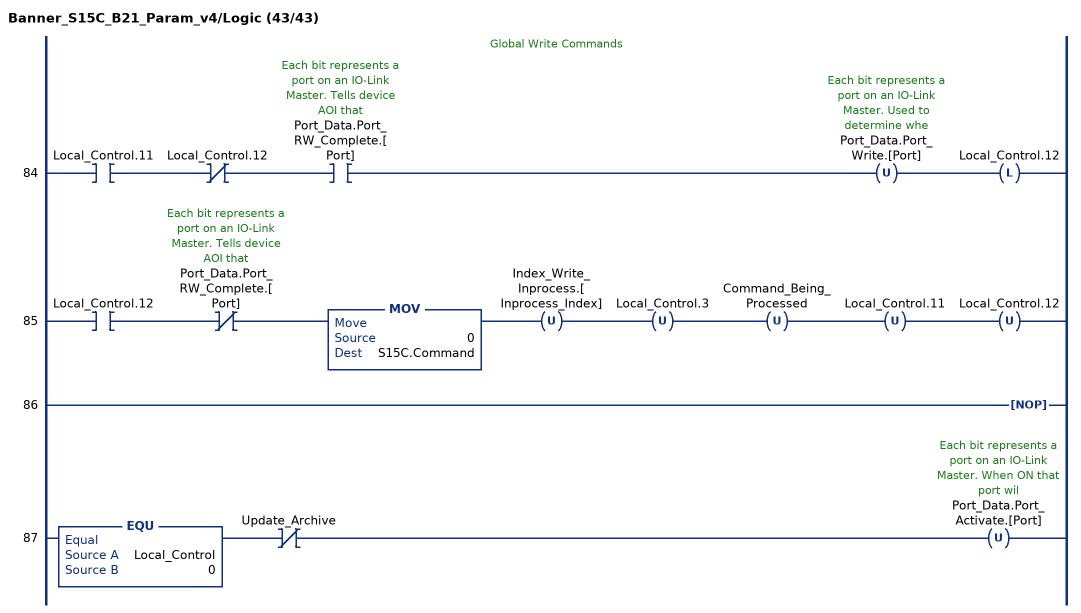
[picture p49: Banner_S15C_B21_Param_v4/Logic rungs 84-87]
   // Global Write Commands
   84: XIC(Local_Control.11)XIO(Local_Control.12)XIC(Port_Data.Port_RW_Complete.[Port])OTU(Port_Data.Port_Write.[Port])OTL(Local_Control.12);
   85: XIC(Local_Control.12)XIO(Port_Data.Port_RW_Complete.[Port])MOV(0,S15C.Command)OTU(Index_Write_Inprocess.[Inprocess_Index])OTU(Local_Control.3)OTU(Command_Being_Processed)OTU(Local_Control.11)OTU(Local_Control.12);
   86: NOP();
   87: EQU(Local_Control,0)XIO(Update_Archive)OTU(Port_Data.Port_Activate.[Port]);
END_ROUTINE
END_ADD_ON_INSTRUCTION
